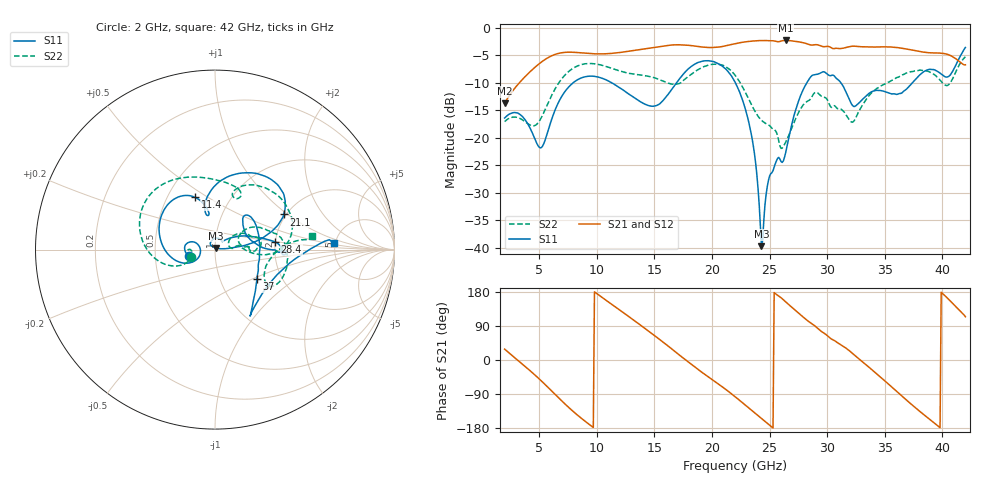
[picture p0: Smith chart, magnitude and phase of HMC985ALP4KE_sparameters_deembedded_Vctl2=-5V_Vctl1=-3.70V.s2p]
!s2p File: Measurements: S11, S21, S12, S22
# GHz S dB R 50.0
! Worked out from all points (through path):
!   401 points, 2 GHz to 42 GHz, reference 50 ohm
!   highest |S21| = -2.30 dB at 26.4 GHz (marker M1); lowest = -13.7 dB at 2 GHz (marker M2)
!   lowest |S11| = -39.7 dB at 24.3 GHz (marker M3), VSWR 1.02, Z = 50.5 + j0.939 ohm
!   |S11| at or under -10 dB: start of sweep to 7.947 GHz; 22.04 GHz to 28.23 GHz (6.198 GHz wide, 24.7 % of centre); 31.19 GHz to 37.4 GHz (6.204 GHz wide, 18.1 % of centre)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
!   |S22| runs from -21.9 to -5.3 dB; largest |S21 - S12| = 0.00079
!   S11 on the Smith chart (normalised r, x): 2 GHz: 0.74, -0.05; 11.4 GHz: 0.68, +0.44; 21.1 GHz: 1.95, +0.94; 28.4 GHz: 1.99, +0.19; 37 GHz: 1.50, -0.53; 42 GHz: 4.85, +0.61
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2  -16.39 -166.9  -13.72 28.6  -13.72 28.7  -17.06 -163.1
3.4  -15.86 168.0  -9.72 -7.3  -9.72 -7.3  -16.55 -180.0
5.1  -21.82 -177.0  -6.38 -52.6  -6.38 -52.6  -16.66 -159.4
6.3  -15.37 -153.6  -4.90 -88.2  -4.90 -88.2  -11.42 -160.8
8.7  -9.08 149.0  -4.57 -154.7  -4.57 -154.7  -6.67 151.8
11.4  -10.12 111.0  -4.63 144.8  -4.63 144.8  -7.44 107.9
13.6  -13.19 100.0  -4.01 96.4  -4.01 96.4  -8.53 77.7
15.4  -13.91 104.0  -3.44 55.5  -3.44 55.5  -9.40 64.5
17.9  -7.56 78.6  -3.17 -4.3  -3.17 -4.2  -8.93 70.8
21.1  -7.32 27.1  -3.32 -75.3  -3.31 -75.3  -6.98 15.7
22  -9.85 17.1  -2.90 -96.7  -2.90 -96.6  -8.61 0.8
23.4  -19.20 6.3  -2.44 -131.5  -2.44 -131.4  -13.85 -4.9
24.3  -39.69 63.8  -2.32 -154.1  -2.32 -154.0  -16.80 5.9
25  -26.95 125.9  -2.35 -171.9  -2.35 -171.8  -17.78 9.6
26.4  -22.68 44.3  -2.30 153.4  -2.30 153.4  -20.79 31.6
28.4  -9.43 7.2  -3.02 101.4  -3.01 101.4  -13.21 18.4
28.7  -8.65 2.1  -3.14 95.3  -3.14 95.3  -12.43 16.8
32.4  -14.30 29.6  -3.35 12.1  -3.34 12.2  -16.71 26.7
35.4  -11.86 16.8  -3.48 -65.7  -3.48 -65.7  -9.82 18.3
37  -10.91 -34.9  -3.90 -108.8  -3.90 -108.7  -8.16 4.3
39.8  -8.24 -55.4  -4.60 -178.7  -4.60 -178.7  -9.51 -32.8
42  -3.58 3.0  -6.72 114.2  -6.72 114.3  -5.26 7.9
